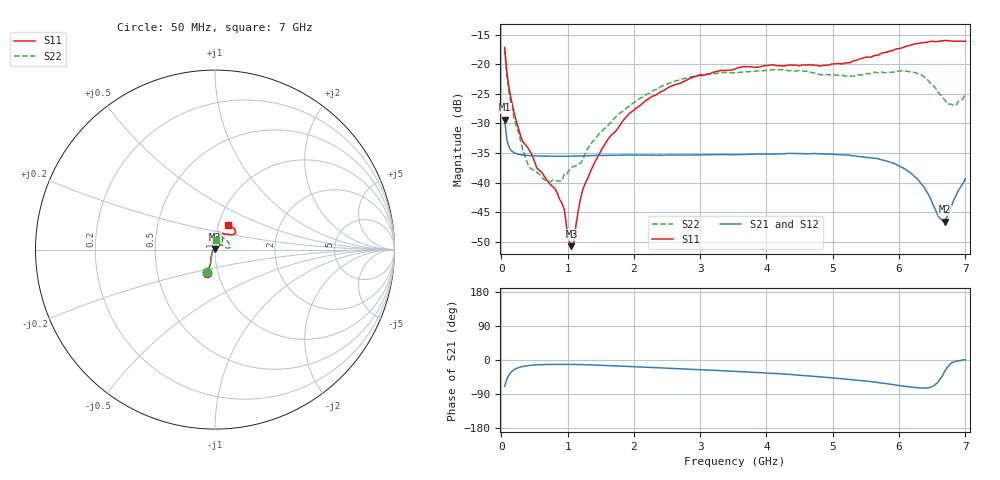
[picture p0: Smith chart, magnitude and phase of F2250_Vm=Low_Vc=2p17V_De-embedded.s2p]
! Integrated Device Technology
! Corporate Headquarters
! 6024 Silver Creek Valley Road
! San Jose, CA 95138  USA
! Phone:  1-408-284-8200
! Toll Free:  1-800-223-1366
! Webpage:  http://www.idt.com/
! Timing and RF Division
! 515 Groton Road, Suite 102
! Westford, MA 01886-6024
! Device:  F2250
! Description: Voltage Variable RF Attenuator
! Frequency:  50.0 -  6000.00 MHz
! Package:  3x3 mm Thin QFN Plastic Package: 16 pin
! Ports:  2 RF, 3 DC
!  Pin  1  = GND
!  Pin  2  = NC
!  Pin  3  = RF1  = Port 1
!  Pin  4  = NC
!  Pin  5  = GND
!  Pin  6  = GND
!  Pin  7  = GND
!  Pin  8  = GND
!  Pin  9  = NC
!  Pin 10  = RF2  = Port 2
!  Pin 11  = NC
!  Pin 12  = GND
!  Pin 13  = GND
!  Pin 14  = VCNTRL
!  Pin 15  = VDD
!  Pin 16  = VMODE
! Vcntrl:  2.170 Volts
! Vmode:  +0.000 Volts
! Vdd:  +3.30  Volts
! Current:  1.180 mA
! Data:  The device was measured on a the F2250 evaluation board which has
!  individual transmission lines to the RF pins.  Data was collected
!  using a calibrated network analyzer.  The evaluation board was
!  de-embedded using a TRL calibration technique.
!  The reference plane is the edge of the package pin.
! Misc:  SN 10
!  Action Tracker AT0258
! Date Measured:  2014-11-26
! Date:  2015-10-15  MJV
! Note:
!  Integrated Device Technology supplies this data as a sample of measured
!  data at the package pin for this product.  Your particular data for this
!  product may vary.
!  Data was taken at 25 degrees C.
!  Integrated Device Technology reserves the right to change this data at anytime.
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# GHz S dB R 50
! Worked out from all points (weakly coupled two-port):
!   201 points, 50 MHz to 7 GHz, reference 50 ohm
!   highest |S21| = -29.37 dB at 50 MHz (marker M1); lowest = -46.6 dB at 6.687 GHz (marker M2)
!   lowest |S11| = -50.8 dB at 1.058 GHz (marker M3), VSWR 1.01, Z = 49.8 + j0.243 ohm
!   |S11| at or under -10 dB: start of sweep to end of sweep
!   |S22| runs from -39.9 to -17.4 dB; largest |S21 - S12| = 5.3e-05
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0.05  -17.18 -108.6  -29.37 -69.3  -29.37 -69.3  -17.44 -110.2
0.08475  -21.44 -107.4  -32.84 -49.9  -32.84 -49.9  -21.98 -108.3
0.189  -28.00 -119.7  -34.95 -26.0  -34.94 -26.0  -29.04 -122.6
0.29325  -32.20 -127.8  -35.31 -18.3  -35.31 -18.3  -33.05 -131.3
0.43225  -34.72 -144.6  -35.46 -14.2  -35.46 -14.2  -37.57 -163.8
0.71025  -39.94 -168.4  -35.55 -11.8  -35.55 -11.8  -39.92 151.8
0.91875  -43.58 158.0  -35.56 -11.6  -35.56 -11.6  -39.64 122.9
0.9535  -44.73 169.9  -35.56 -11.6  -35.56 -11.6  -38.50 121.3
1.023  -50.07 144.1  -35.55 -11.6  -35.55 -11.6  -37.99 103.6
1.05775  -50.76 122.8  -35.55 -11.7  -35.55 -11.7  -37.43 98.7
1.0925  -50.32 89.6  -35.53 -11.8  -35.54 -11.8  -37.31 93.8
1.162  -44.71 56.4  -35.52 -12.0  -35.52 -12.0  -36.86 82.3
1.2315  -41.12 44.3  -35.49 -12.2  -35.49 -12.2  -36.13 73.2
1.6485  -32.12 42.0  -35.40 -14.8  -35.40 -14.8  -29.87 58.2
2.37825  -24.87 47.4  -35.36 -20.5  -35.37 -20.5  -24.05 53.7
3.525  -20.80 72.5  -35.30 -29.8  -35.30 -29.8  -21.45 73.2
4.7065  -20.17 72.4  -35.10 -42.9  -35.11 -42.9  -21.46 71.4
5.85325  -17.81 40.4  -36.53 -63.5  -36.52 -63.6  -21.34 21.3
6.27025  -16.50 40.1  -39.34 -72.8  -39.35 -72.8  -21.54 8.0
6.68725  -15.99 48.8  -46.63 -30.0  -46.58 -29.6  -26.04 27.1
6.82625  -16.14 53.6  -42.94 -5.3  -42.91 -5.0  -27.04 52.8
7  -16.12 63.2  -39.34 0.5  -39.30 0.4  -24.96 84.2
